| IBIS file stm32n657_vfbga223.ibs
[IBIS ver] 4.2
[File name] stm32n657_vfbga223.ibs
[File Rev] 1.0
[Date] 20-09-2024
[Source] Data Created at STMicroelectronics
[Notes]  File originated from ELDO simulations.
[Disclaimer]  This information is for modeling purpose only and is
   not guaranteed. The information is subject to change without
   notice.
[Copyright] Copyright 2024 STMicroelectronics Inc.
|   Component stm32n657_vfbga223
[Component] stm32n657_vfbga223
[Manufacturer] STMicroelectronics
[Package]
| variable   typ   min   max
R_pkg  0  NA  NA
L_pkg  0  NA  NA
C_pkg  0  NA  NA
[Pin]   signal_name   model_name
A1  PDR_ON  nc
A2  OTG1_TXRTUNE  nc
A3  OTG1_HSDP  USB2_HS_IBIS
A4  UCPD1_CC1  nc
A5  PH0-OSC_IN  isudq_tt
A6  PC12  io8_tt
A7  PC1  io8_tt_i3c
A8  PC6  io8_tt
A9  PE13  io8_tt_i3c
A10  PD6  io8_tt
A11  PD12  io8_tt
A12  PD15  io8_tt_i3c
A13  PE8  io8_tt
A14  PB15  io8_tt
A15  PD5  io8_tt
A16  PB13  io8_tt
A17  PD11  io8_tt_i3c
A18  PE0  io8_tt
A19  VSS  gnd
B1  NC  nc
B2  OTG1_ID  nc
B3  OTG1_HSDM  USB2_HS_IBIS
B4  UCPD1_CC2  nc
B5  PH1-OSC_OUT  isudq_tt
B6  PC11  io8_tt_i3c
B7  PH9  io8_tt_i3c
B8  PC7  io8_tt
B9  PE6  io8_tt_i3c
B10  PD2  io8_tt
B11  PE7  io8_tt
B12  PD0  io8_tt
B13  PD4  io8_tt_i3c
B14  PD8  io8_tt
B15  PB9  io8_tt
B16  PB2  io8_tt
B17  PB3  io8_tt
B18  PE1  io8_tt
B19  PE2  io8_tt
C1  OTG2_HSDP  USB2_HS_IBIS
C2  OTG2_HSDM  USB2_HS_IBIS
C3  VDD33USB  power
C17  PB14  io8_tt
C18  PE3  io8_tt
C19  PB0  io8_tt
D1  PC15-OSC32_OUT  io8_tt_sw
D2  NC  nc
D4  VDDA18USB  power
D5  PC9  io8_tt_i3c
D6  PC10  io8_tt_i3c
D7  PH2  io8_tt
D8  PE11  io8_tt
D9  PE5  io8_tt_i3c
D10  PE12  io8_tt
D11  PD10  io8_tt
D12  PD1  io8_tt
D13  PD3  io8_tt_i3c
D14  PE10  io8_tt
D15  PB8  io8_tt
D16  PD13  io8_tt
D18  PP10  io8_tt
D19  PB6  io8_tt
E1  PC14-OSC32_IN  io8_tt_sw
E2  OTG2_TXRTUNE  nc
E4  OTG2_ID  nc
E16  PB7  io8_tt
E18  PO3  io8_tt
E19  PP9  io8_tt
F1  VBAT  power
F2  NRST  ioreset_tt_v18_1v8
F4  BOOT0  isudq_tt
F6  PC8  io8_tt_i3c
F7  VDDIO4  power
F8  VDDIO4  power
F9  PE14  io8_tt_i3c
F10  PE15  io8_tt_i3c
F11  PD7  io8_tt
F12  VSS  gnd
F13  PD14  io8_tt_i3c
F14  PE9  io8_tt
F16  PO0  io8_tt
F18  PP1  io8_tt
F19  PP8  io8_tt
G1  V08CAP  nc
G2  VFBSMPS  nc
G4  PWR_ON  io8_tt
G6  VSSAON  nc
G14  PD9  io8_tt
G16  PO5  io8_tt
G18  PO2  io8_tt
G19  PP7  io8_tt
H1  VDDA18PMU  nc
H2  VSSAPMU  nc
H4  PC13  io8_tt_tamp
H6  VDDA18AON  nc
H14  VSS  gnd
H16  VDDIO2  power
H18  PP0  io8_tt
H19  PP6  io8_tt
J1  VSSSMPS  nc
J2  VSSSMPS  nc
J3  VSSSMPS  nc
J4  VSSSMPS  nc
J5  VSSSMPS  nc
J14  VDD  power
J16  VDDIO2  power
J18  PO4  io8_tt
J19  PP5  io8_tt
K1  VLXSMPS  nc
K2  VLXSMPS  nc
K3  VLXSMPS  nc
K4  VLXSMPS  nc
K5  VLXSMPS  nc
K14  VDD  power
K16  VDDIO2  power
K18  PP2  io8_tt
K19  PP3  io8_tt
L1  VDDSMPS  nc
L2  VDDSMPS  nc
L3  VDDSMPS  nc
L4  VDDSMPS  nc
L5  VDDSMPS  nc
L14  VDD  power
L16  VDDIO2  power
L18  PP15  io8_tt
L19  PP4  io8_tt
M1  PF4  io8_tt
M2  PF10  io8_tt
M4  PF6  io8_tt
M6  VDDA18PLL  nc
M14  VDDIO3  power
M16  VDDIO3  power
M18  PP14  io8_tt
M19  PP13  io8_tt
N1  PG6  io8_tt
N2  PG5  io8_tt
N4  PF5  io8_tt
N6  VSSA  nc
N14  PO1  io8_tt
N16  VSS  gnd
N18  PP12  io8_tt
N19  PP11  io8_tt
P1  PF3  io8_tt
P2  PF14  io8_tt
P4  PF2  io8_tt
P6  VDDA18ADC  nc
P7  VDDCORE  nc
P8  VSS  gnd
P9  VDDCORE  nc
P10  VDDCORE  nc
P11  VDDCORE  nc
P12  VSS  gnd
P13  VDDCORE  nc
P14  VSS  gnd
P16  PN1  io8_tt
P18  PN11  io8_tt
P19  PN3  io8_tt
R1  PF15  io8_tt
R2  PF7  io8_tt
R4  PF8  io8_tt
R16  PN7  io8_tt
R18  PN10  io8_tt
R19  PN0  io8_tt
T1  PF11  io8_tt
T2  PF9  io8_tt
T4  PG4  io8_tt
T5  PG3  io8_tt
T6  CSI_REXT  nc
T7  PG14  io8_tt
T8  PA11  io8_tt
T9  PA8  io8_tt_i3c
T10  PA6  io8_tt_i3c
T11  PG1  io8_tt
T12  PG10  io8_tt
T13  PB10  io8_tt_i3c
T14  PB5  io8_tt_i3c
T15  PA15  io8_tt
T16  PG0  io8_tt
T18  PN9  io8_tt
T19  PN2  io8_tt
U1  PF1  io8_tt
U2  PF12  io8_tt
U3  PF0  io8_tt
U17  PA3  io8_tt
U18  PN5  io8_tt
U19  PN6  io8_tt
V1  PF13  io8_tt
V2  VREFM  nc
V3  CSI_D1N  DPHY_IBIS_L1
V4  CSI_CKN  DPHY_IBIS_L1
V5  CSI_D0N  DPHY_IBIS_L1
V6  VDDA18CSI  power
V7  PA14  io8_tt
V8  PA12  io8_tt
V9  PA9  io8_tt_i3c
V10  PA5  io8_tt_i3c
V11  PG12  io8_tt
V12  PA0  io8_tt
V13  PB11  io8_tt_i3c
V14  PB1  io8_tt
V15  PA7  io8_tt
V16  PG9  io8_tt
V17  PG8  io8_tt
V18  PN8  io8_tt
V19  PN4  io8_tt
W1  VSS  gnd
W2  VREFP  nc
W3  CSI_D1P  DPHY_IBIS_L1
W4  CSI_CKP  DPHY_IBIS_L1
W5  CSI_D0P  DPHY_IBIS_L1
W6  VDDCSI  nc
W7  PA13  io8_tt
W8  PG15  io8_tt
W9  PA10  io8_tt
W10  PA2  io8_tt
W11  PG13  io8_tt
W12  PA1  io8_tt
W13  PB12  io8_tt_i3c
W14  PG2  io8_tt
W15  PB4  io8_tt
W16  PG11  io8_tt
W17  PA4  io8_tt
W18  PN12  io8_tt
W19  VSS  gnd
[Package Model]   486-fcvfbga-10x10-223-240119
[Pin Mapping]   pulldown_ref   pullup_ref   | Comment
A1  nc  nc
A2  nc  nc
A3  gnd  VDD33USB
A4  nc  nc
A5  gnd  VDD
A6  gnd  VDDIO4
A7  gnd  VDDIO4
A8  gnd  VDDIO4
A9  gnd  VDD
A10  gnd  VDD
A11  gnd  VDD
A12  gnd  VDD
A13  gnd  VDD
A14  gnd  VDD
A15  gnd  VDD
A16  gnd  VDD
A17  gnd  VDD
A18  gnd  VDD
A19  gnd  nc
B1  nc  nc
B2  nc  nc
B3  gnd  VDD33USB
B4  nc  nc
B5  gnd  VDD
B6  gnd  VDDIO4
B7  gnd  VDDIO4
B8  gnd  VDDIO4
B9  gnd  VDD
B10  gnd  VDD
B11  gnd  VDD
B12  gnd  VDD
B13  gnd  VDD
B14  gnd  VDD
B15  gnd  VDD
B16  gnd  VDD
B17  gnd  VDD
B18  gnd  VDD
B19  gnd  VDD
C1  gnd  VDD33USB
C2  gnd  VDD33USB
C3  nc  VDD33USB
C17  gnd  VDD
C18  gnd  VDD
C19  gnd  VDD
D1  gnd  VSW
D2  nc  nc
D4  nc  VDDA18USB
D5  gnd  VDDIO4
D6  gnd  VDDIO4
D7  gnd  VDDIO4
D8  gnd  VDD
D9  gnd  VDD
D10  gnd  VDD
D11  gnd  VDD
D12  gnd  VDD
D13  gnd  VDD
D14  gnd  VDD
D15  gnd  VDD
D16  gnd  VDD
D18  gnd  VDDIO2
D19  gnd  VDD
E1  gnd  VSW
E2  nc  nc
E4  nc  nc
E16  gnd  VDD
E18  gnd  VDDIO2
E19  gnd  VDDIO2
F1  nc  VSW
F2  gnd  VDD
F4  gnd  VDD
F6  gnd  VDDIO4
F7  nc  VDDIO4
F8  nc  VDDIO4
F9  gnd  VDD
F10  gnd  VDD
F11  gnd  VDD
F12  gnd  nc
F13  gnd  VDD
F14  gnd  VDD
F16  gnd  VDDIO2
F18  gnd  VDDIO2
F19  gnd  VDDIO2
G1  nc  nc
G2  nc  nc
G4  gnd  VDD
G6  nc  nc
G14  gnd  VDD
G16  gnd  VDDIO2
G18  gnd  VDDIO2
G19  gnd  VDDIO2
H1  nc  nc
H2  nc  nc
H4  gnd  VSW
H6  nc  nc
H14  gnd  nc
H16  nc  VDDIO2
H18  gnd  VDDIO2
H19  gnd  VDDIO2
J1  nc  nc
J2  nc  nc
J3  nc  nc
J4  nc  nc
J5  nc  nc
J14  nc  VDD
J16  nc  VDDIO2
J18  gnd  VDDIO2
J19  gnd  VDDIO2
K1  nc  nc
K2  nc  nc
K3  nc  nc
K4  nc  nc
K5  nc  nc
K14  nc  VDD
K16  nc  VDDIO2
K18  gnd  VDDIO2
K19  gnd  VDDIO2
L1  nc  nc
L2  nc  nc
L3  nc  nc
L4  nc  nc
L5  nc  nc
L14  nc  VDD
L16  nc  VDDIO2
L18  gnd  VDDIO2
L19  gnd  VDDIO2
M1  gnd  VDD
M2  gnd  VDD
M4  gnd  VDD
M6  nc  nc
M14  nc  VDDIO3
M16  nc  VDDIO3
M18  gnd  VDDIO2
M19  gnd  VDDIO2
N1  gnd  VDD
N2  gnd  VDD
N4  gnd  VDD
N6  nc  nc
N14  gnd  VDDIO2
N16  gnd  nc
N18  gnd  VDDIO2
N19  gnd  VDDIO2
P1  gnd  VDD
P2  gnd  VDD
P4  gnd  VDD
P6  nc  nc
P7  nc  nc
P8  gnd  nc
P9  nc  nc
P10  nc  nc
P11  nc  nc
P12  gnd  nc
P13  nc  nc
P14  gnd  nc
P16  gnd  VDDIO3
P18  gnd  VDDIO3
P19  gnd  VDDIO3
R1  gnd  VDD
R2  gnd  VDD
R4  gnd  VDD
R16  gnd  VDDIO3
R18  gnd  VDDIO3
R19  gnd  VDDIO3
T1  gnd  VDD
T2  gnd  VDD
T4  gnd  VDD
T5  gnd  VDD
T6  nc  nc
T7  gnd  VDD
T8  gnd  VDD
T9  gnd  VDD
T10  gnd  VDD
T11  gnd  VDD
T12  gnd  VDD
T13  gnd  VDD
T14  gnd  VDD
T15  gnd  VDD
T16  gnd  VDD
T18  gnd  VDDIO3
T19  gnd  VDDIO3
U1  gnd  VDD
U2  gnd  VDD
U3  gnd  VDD
U17  gnd  VDD
U18  gnd  VDDIO3
U19  gnd  VDDIO3
V1  gnd  VDD
V2  nc  nc
V3  gnd  VDDA18CSI
V4  gnd  VDDA18CSI
V5  gnd  VDDA18CSI
V6  nc  VDDA18CSI
V7  gnd  VDD
V8  gnd  VDD
V9  gnd  VDD
V10  gnd  VDD
V11  gnd  VDD
V12  gnd  VDD
V13  gnd  VDD
V14  gnd  VDD
V15  gnd  VDD
V16  gnd  VDD
V17  gnd  VDD
V18  gnd  VDDIO3
V19  gnd  VDDIO3
W1  gnd  nc
W2  nc  nc
W3  gnd  VDDA18CSI
W4  gnd  VDDA18CSI
W5  gnd  VDDA18CSI
W6  nc  nc
W7  gnd  VDD
W8  gnd  VDD
W9  gnd  VDD
W10  gnd  VDD
W11  gnd  VDD
W12  gnd  VDD
W13  gnd  VDD
W14  gnd  VDD
W15  gnd  VDD
W16  gnd  VDD
W17  gnd  VDD
W18  gnd  VDDIO3
W19  gnd  nc
[Diff Pin]   inv_pin   vdiff   tdelay_typ   tdelay_min   tdelay_max
W4   V4   NA   NA   NA   NA
W5   V5   NA   NA   NA   NA
W3   V3   NA   NA   NA   NA
A3   B3   NA   NA   NA   NA
C1   C2   NA   NA   NA   NA
[Model Selector] DPHY_IBIS_L1
DPHY_RX_2P5G_L1   DPHY HSRX model at 2.5Gbps for lane 1
DPHY_RX_1P5G_L1   DPHY HSRX model at 1.5Gbps for lane 1
[Model Selector] io8_tt
io8_tt_ls_3v3 "GPIO - 3V tolerant - low speed - 3.3V range"
io8_tt_ms_3v3 "GPIO - 3V tolerant - med speed - 3.3V range"
io8_tt_fs_3v3 "GPIO - 3V tolerant - fast speed - 3.3V range"
io8_tt_hs_3v3 "GPIO - 3V tolerant - high speed - 3.3V range"
io8_tt_hslv_ls_1v8 "GPIO low voltage optimization - 3V tolerant - low speed - 1.8V range"
io8_tt_hslv_ms_1v8 "GPIO low voltage optimization - 3V tolerant - med speed - 1.8V range"
io8_tt_hslv_fs_1v8 "GPIO low voltage optimization - 3V tolerant - fast speed - 1.8V range"
io8_tt_hslv_hs_1v8 "GPIO low voltage optimization - 3V tolerant - high speed - 1.8V range"
[Model Selector] io8_tt_i3c
io8_tt_ls_3v3 "GPIO - 3V tolerant - low speed - 3.3V range"
io8_tt_ms_3v3 "GPIO - 3V tolerant - med speed - 3.3V range"
io8_tt_fs_3v3 "GPIO - 3V tolerant - fast speed - 3.3V range"
io8_tt_hs_3v3 "GPIO - 3V tolerant - high speed - 3.3V range"
io8_tt_hslv_ls_1v8 "GPIO low voltage optimization - 3V tolerant - low speed - 1.8V range"
io8_tt_hslv_ms_1v8 "GPIO low voltage optimization - 3V tolerant - med speed - 1.8V range"
io8_tt_hslv_fs_1v8 "GPIO low voltage optimization - 3V tolerant - fast speed - 1.8V range"
io8_tt_hslv_hs_1v8 "GPIO low voltage optimization - 3V tolerant - high speed - 1.8V range"
io8_tt_i3c_ls_3v3 "GPIO with I3C open-drain - 3V tolerant - low speed - 3.3V range"
io8_tt_i3c_ms_3v3 "GPIO with I3C open-drain - 3V tolerant - med speed - 3.3V range"
io8_tt_i3c_fs_3v3 "GPIO with I3C open-drain - 3V tolerant - fast speed - 3.3V range"
io8_tt_i3c_hs_3v3 "GPIO with I3C open-drain - 3V tolerant - high speed - 3.3V range"
io8_tt_hslv_i3c_ls_1v8 "GPIO low voltage optimization with I3C open-drain - 3V tolerant - low speed - 1.8V range"
io8_tt_hslv_i3c_ms_1v8 "GPIO low voltage optimization with I3C open-drain - 3V tolerant - med speed - 1.8V range"
io8_tt_hslv_i3c_fs_1v8 "GPIO low voltage optimization with I3C open-drain - 3V tolerant - fast speed - 1.8V range"
io8_tt_hslv_i3c_hs_1v8 "GPIO low voltage optimization with I3C open-drain - 3V tolerant - high speed - 1.8V range"
io8_tt_i3c_fmp_3v3 "GPIO with I3C fm+ open-drain - 3V tolerant - 3.3V range"
[Model Selector] io8_tt_sw
io8_tt_sw_3v3 "Input Buffer - 3V tolerant - 3.3V range"
io8_tt_sw_1v8 "Input Buffer - 3V tolerant - 1.8V range"
[Model Selector] io8_tt_tamp
io8_tt_ls_3v3 "GPIO - 3V tolerant - low speed - 3.3V range"
io8_tt_ms_3v3 "GPIO - 3V tolerant - med speed - 3.3V range"
io8_tt_fs_3v3 "GPIO - 3V tolerant - fast speed - 3.3V range"
io8_tt_hs_3v3 "GPIO - 3V tolerant - high speed - 3.3V range"
io8_tt_hslv_ls_1v8 "GPIO low voltage optimization - 3V tolerant - low speed - 1.8V range"
io8_tt_hslv_ms_1v8 "GPIO low voltage optimization - 3V tolerant - med speed - 1.8V range"
io8_tt_hslv_fs_1v8 "GPIO low voltage optimization - 3V tolerant - fast speed - 1.8V range"
io8_tt_hslv_hs_1v8 "GPIO low voltage optimization - 3V tolerant - high speed - 1.8V range"
io8_tt_tamp_3v3 "IO tamper - 3V tolerant - 3.3V range"
io8_tt_tamp_1v8 "IO tamper - 3V tolerant - 1.8V range"
|[Model Selector] ioreset_tt_v18
|ioreset_tt_v18_1v8 "Reset PAD - 3V tolerant - 1.8V range"
[Model Selector] isudq_tt
isudq_tt_3v3 "Input Buffer - 3V tolerant - 3.3V range"
isudq_tt_1v8 "Input Buffer - 3V tolerant - 1.8V range"
[Model Selector] USB2_HS_IBIS
USB2_HSRX   USB2 HSRX model
USB2_HSTX_00_0_01_0011_11   TuningBits_AMP_PULSE_RISE_REF_XV=00_0_01_0011_11
USB2_HSTX_00_0_10_0101_11   TuningBits_AMP_PULSE_RISE_REF_XV=00_0_10_0101_11
USB2_HSTX_00_0_11_0111_11   TuningBits_AMP_PULSE_RISE_REF_XV=00_0_11_0111_11
USB2_HSTX_00_1_01_0011_11   TuningBits_AMP_PULSE_RISE_REF_XV=00_1_01_0011_11
USB2_HSTX_00_1_10_0101_11   TuningBits_AMP_PULSE_RISE_REF_XV=00_1_10_0101_11
USB2_HSTX_00_1_11_0111_11   TuningBits_AMP_PULSE_RISE_REF_XV=00_1_11_0111_11
USB2_HSTX_01_0_01_0011_11   TuningBits_AMP_PULSE_RISE_REF_XV=01_0_01_0011_11
USB2_HSTX_01_0_10_0101_11   TuningBits_AMP_PULSE_RISE_REF_XV=01_0_10_0101_11
USB2_HSTX_01_0_11_0111_11   TuningBits_AMP_PULSE_RISE_REF_XV=01_0_11_0111_11
USB2_HSTX_01_1_01_0011_11   TuningBits_AMP_PULSE_RISE_REF_XV=01_1_01_0011_11
USB2_HSTX_01_1_10_0101_11   TuningBits_AMP_PULSE_RISE_REF_XV=01_1_10_0101_11
USB2_HSTX_01_1_11_0111_11   TuningBits_AMP_PULSE_RISE_REF_XV=01_1_11_0111_11
USB2_HSTX_10_0_01_0011_11   TuningBits_AMP_PULSE_RISE_REF_XV=10_0_01_0011_11
USB2_HSTX_10_0_10_0101_11   TuningBits_AMP_PULSE_RISE_REF_XV=10_0_10_0101_11
USB2_HSTX_10_0_11_0111_11   TuningBits_AMP_PULSE_RISE_REF_XV=10_0_11_0111_11
USB2_HSTX_10_1_01_0011_11   TuningBits_AMP_PULSE_RISE_REF_XV=10_1_01_0011_11
USB2_HSTX_10_1_10_0101_11   TuningBits_AMP_PULSE_RISE_REF_XV=10_1_10_0101_11
USB2_HSTX_10_1_11_0111_11   TuningBits_AMP_PULSE_RISE_REF_XV=10_1_11_0111_11
[Define Package Model]  486-fcvfbga-10x10-223-240119
[Manufacturer]  unknown
[OEM]  unknown
[Description]  unknown
[Number Of Pins]  192
[Pin Numbers]
| Pin Name Terminal   Net Name   Starting Node   Ending Node
F4 | BOOT0
V4 | CSI_CKN
W4 | CSI_CKP
V5 | CSI_D0N
W5 | CSI_D0P
V3 | CSI_D1N
W3 | CSI_D1P
T6 | CSI_REXT
F2 | NRST
B3 | OTG1_HSDM
A3 | OTG1_HSDP
B2 | OTG1_ID
A2 | OTG1_TXRTUNE
B1 | NC
C2 | OTG2_HSDM
C1 | OTG2_HSDP
E4 | OTG2_ID
E2 | OTG2_TXRTUNE
D2 | NC
V12 | PA0
W12 | PA1
W10 | PA2
U17 | PA3
W17 | PA4
V10 | PA5
T10 | PA6
V15 | PA7
T9 | PA8
V9 | PA9
W9 | PA10
T8 | PA11
V8 | PA12
W7 | PA13
V7 | PA14
T15 | PA15
C19 | PB0
V14 | PB1
B16 | PB2
B17 | PB3
W15 | PB4
T14 | PB5
D19 | PB6
E16 | PB7
D15 | PB8
B15 | PB9
T13 | PB10
V13 | PB11
W13 | PB12
A16 | PB13
C17 | PB14
A14 | PB15
A7 | PC1
A8 | PC6
B8 | PC7
F6 | PC8
D5 | PC9
D6 | PC10
B6 | PC11
A6 | PC12
H4 | PC13
E1 | PC14-OSC32_IN
D1 | PC15-OSC32_OUT
B12 | PD0
D12 | PD1
B10 | PD2
D13 | PD3
B13 | PD4
A15 | PD5
A10 | PD6
F11 | PD7
B14 | PD8
G14 | PD9
D11 | PD10
A17 | PD11
A11 | PD12
D16 | PD13
F13 | PD14
A12 | PD15
A1 | PDR_ON
A18 | PE0
B18 | PE1
B19 | PE2
C18 | PE3
D9 | PE5
B9 | PE6
B11 | PE7
A13 | PE8
F14 | PE9
D14 | PE10
D8 | PE11
D10 | PE12
A9 | PE13
F9 | PE14
F10 | PE15
U3 | PF0
U1 | PF1
P4 | PF2
P1 | PF3
M1 | PF4
N4 | PF5
M4 | PF6
R2 | PF7
R4 | PF8
T2 | PF9
M2 | PF10
T1 | PF11
U2 | PF12
V1 | PF13
P2 | PF14
R1 | PF15
T16 | PG0
T11 | PG1
W14 | PG2
T5 | PG3
T4 | PG4
N2 | PG5
N1 | PG6
V17 | PG8
V16 | PG9
T12 | PG10
W16 | PG11
V11 | PG12
W11 | PG13
T7 | PG14
W8 | PG15
A5 | PH0-OSC_IN
B5 | PH1-OSC_OUT
D7 | PH2
B7 | PH9
R19 | PN0
P16 | PN1
T19 | PN2
P19 | PN3
V19 | PN4
U18 | PN5
U19 | PN6
R16 | PN7
V18 | PN8
T18 | PN9
R18 | PN10
P18 | PN11
W18 | PN12
F16 | PO0
N14 | PO1
G18 | PO2
E18 | PO3
J18 | PO4
G16 | PO5
H18 | PP0
F18 | PP1
K18 | PP2
K19 | PP3
L19 | PP4
J19 | PP5
H19 | PP6
G19 | PP7
F19 | PP8
E19 | PP9
D18 | PP10
N19 | PP11
N18 | PP12
M19 | PP13
M18 | PP14
L18 | PP15
G4 | PWR_ON
A4 | UCPD1_CC1
B4 | UCPD1_CC2
G1 | V08CAP
F1 | VBAT
C3 | VDD33USB
J14 | VDD
P6 | VDDA18ADC
H6 | VDDA18AON
V6 | VDDA18CSI
M6 | VDDA18PLL
H1 | VDDA18PMU
D4 | VDDA18USB
P7 | VDDCORE
W6 | VDDCSI
H16 | VDDIO2
M14 | VDDIO3
F7 | VDDIO4
L1 | VDDSMPS
G2 | VFBSMPS
K1 | VLXSMPS
V2 | VREFM
W2 | VREFP
A19 | VSS
N6 | VSSA
G6 | VSSAON
H2 | VSSAPMU
J1 | VSSSMPS
|[Merged Pins]  J14
|K14  |  VDD
|L14  |  VDD
|[Merged Pins]  P7
|P9  |  VDDCORE
|P10  |  VDDCORE
|P11  |  VDDCORE
|P13  |  VDDCORE
|[Merged Pins]  H16
|J16  |  VDDIO2
|K16  |  VDDIO2
|L16  |  VDDIO2
|[Merged Pins]  M14
|M16  |  VDDIO3
|[Merged Pins]  F7
|F8  |  VDDIO4
|[Merged Pins]  L1
|L2  |  VDDSMPS
|L3  |  VDDSMPS
|L4  |  VDDSMPS
|L5  |  VDDSMPS
|[Merged Pins]  K1
|K2  |  VLXSMPS
|K3  |  VLXSMPS
|K4  |  VLXSMPS
|K5  |  VLXSMPS
|[Merged Pins]  A19
|F12  |  VSS
|H14  |  VSS
|N16  |  VSS
|P8  |  VSS
|P12  |  VSS
|P14  |  VSS
|W1  |  VSS
|W19  |  VSS
|[Merged Pins]  J1
|J2  |  VSSSMPS
|J3  |  VSSSMPS
|J4  |  VSSSMPS
|J5  |  VSSSMPS
[Model Data]
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[End Model Data]
[End Package Model]
|End [Component]
| Models and submodels in the file (45): DPHY_RX_1P5G_L1 (Input), DPHY_RX_2P5G_L1 (Input), io8_tt_fs_3v3 (I/O), io8_tt_hs_3v3 (I/O), io8_tt_hslv_fs_1v8 (I/O), io8_tt_hslv_hs_1v8 (I/O), io8_tt_hslv_i3c_fs_1v8 (I/O_open_drain), io8_tt_hslv_i3c_hs_1v8 (I/O_open_drain), io8_tt_hslv_i3c_ls_1v8 (I/O_open_drain), io8_tt_hslv_i3c_ms_1v8 (I/O_open_drain), io8_tt_hslv_ls_1v8 (I/O), io8_tt_hslv_ms_1v8 (I/O), io8_tt_i3c_fmp_3v3 (I/O_open_drain), io8_tt_i3c_fs_3v3 (I/O_open_drain), io8_tt_i3c_hs_3v3 (I/O_open_drain), io8_tt_i3c_ls_3v3 (I/O_open_drain), io8_tt_i3c_ms_3v3 (I/O_open_drain), io8_tt_ls_3v3 (I/O), io8_tt_ms_3v3 (I/O), io8_tt_sw_1v8 (I/O), io8_tt_sw_3v3 (I/O), io8_tt_tamp_1v8 (I/O), io8_tt_tamp_3v3 (I/O), ioreset_tt_v18_1v8 (I/O_open_drain), isudq_tt_1v8 (Input), isudq_tt_3v3 (Input), USB2_HSRX (Input), USB2_HSTX_00_0_01_0011_11 (Output), USB2_HSTX_00_0_10_0101_11 (Output), USB2_HSTX_00_0_11_0111_11 (Output), USB2_HSTX_00_1_01_0011_11 (Output), USB2_HSTX_00_1_10_0101_11 (Output), USB2_HSTX_00_1_11_0111_11 (Output), USB2_HSTX_01_0_01_0011_11 (Output), USB2_HSTX_01_0_10_0101_11 (Output), USB2_HSTX_01_0_11_0111_11 (Output), USB2_HSTX_01_1_01_0011_11 (Output), USB2_HSTX_01_1_10_0101_11 (Output), USB2_HSTX_01_1_11_0111_11 (Output), USB2_HSTX_10_0_01_0011_11 (Output), USB2_HSTX_10_0_10_0101_11 (Output), USB2_HSTX_10_0_11_0111_11 (Output), USB2_HSTX_10_1_01_0011_11 (Output), USB2_HSTX_10_1_10_0101_11 (Output), USB2_HSTX_10_1_11_0111_11 (Output)
